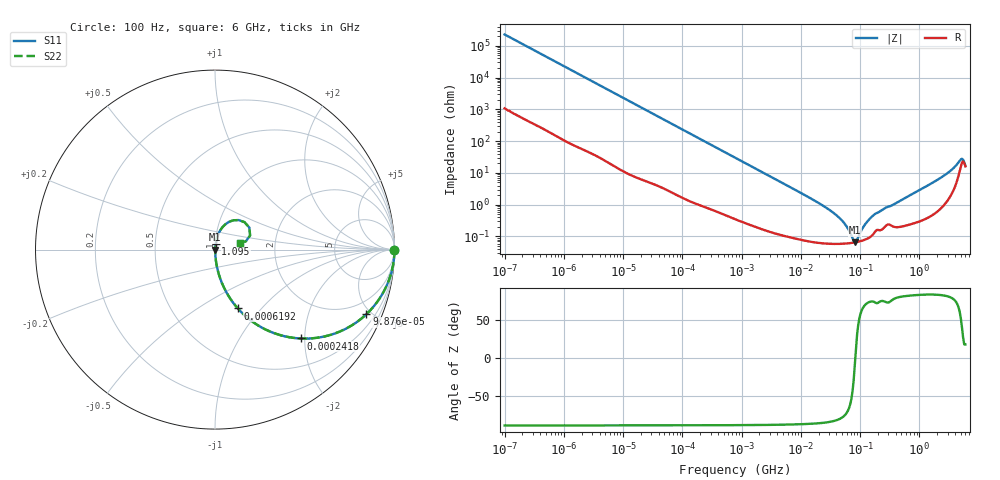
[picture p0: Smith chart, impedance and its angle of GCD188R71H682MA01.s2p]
!Murata Part Number: GCD188R71H682MA01
!These Parameters are Measured in Series Mode Connection
!Data Generated on Mar 13, 2026
!  o--ll--o
!Port1  Port2
!  o------o
!Operation Temp=25[degC], DC Bias Voltage=0[V]
!Freq. Start=100[Hz] Stop=6[GHz] 401[Steps]
# Hz S RI R 50
!Freq.(Hz) S11(Real) S11(Imag) S21(Real) S21(Imag) S12(Real) S12(Imag) S22(Real) S22(Imag)
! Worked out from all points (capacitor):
!   401 points, 100 Hz to 6 GHz, reference 50 ohm
!   read as one part in series: C = 7.03 nF near 109 Hz
!   lowest |Z| = 65.9 mohm at 81.54 MHz (marker M1)
!   series resonance near 83.08 MHz, so ESL is about 520 pH
!   S11 on the Smith chart (normalised r, x): 100 Hz: open; 98.76 kHz: 1.03, -4.68; 241.8 kHz: 1.02, -1.92; 619.2 kHz: 1.01, -0.75; 1.095 GHz: 1.01, +0.06; 6 GHz: 1.32, +0.10
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100  1 -0.000442  2.3e-06 0.000442  2.3e-06 0.000442  1 -0.000442
2008  0.9999 -0.0088  0.000121 0.0088  0.000121 0.0088  0.9999 -0.0088
12592  0.9967 -0.0547  0.00327 0.0547  0.00327 0.0547  0.9967 -0.0547
40335  0.9692 -0.1695  0.0308 0.1695  0.0308 0.1695  0.9692 -0.1695
98762  0.844 -0.3593  0.156 0.3593  0.156 0.3593  0.844 -0.3593
241822  0.4797 -0.4953  0.5203 0.4953  0.5203 0.4953  0.4797 -0.4953
619225  0.1271 -0.3277  0.8729 0.3277  0.8729 0.3277  0.1271 -0.3277
774597  0.0861 -0.2748  0.9139 0.2748  0.9139 0.2748  0.0861 -0.2748
2594782  0.00965 -0.0897  0.9903 0.0897  0.9903 0.0897  0.00965 -0.0897
1.555665e7  0.00089 -0.0148  0.9991 0.0148  0.9991 0.0148  0.00089 -0.0148
4.556224e7  0.000599 -0.00368  0.9994 0.00368  0.9994 0.00368  0.000599 -0.00368
5.960426e7  0.000606 -0.00195  0.9994 0.00195  0.9994 0.00195  0.000606 -0.00195
8.154455e7  0.00065 -0.000106  0.9994 0.000106  0.9994 0.000106  0.00065 -0.000106
8.918374e7  0.000672 0.000412  0.9993 -0.000412  0.9993 -0.000412  0.000672 0.000412
1.166697e8  0.000776 0.00201  0.9992 -0.00201  0.9992 -0.00201  0.000776 0.00201
1.526266e8  0.00102 0.00379  0.999 -0.00379  0.999 -0.00379  0.00102 0.00379
3.124326e8  0.00243 0.00844  0.9976 -0.00844  0.9976 -0.00844  0.00243 0.00844
1.094528e9  0.0041 0.031  0.9959 -0.031  0.9959 -0.031  0.0041 0.031
3.352442e9  0.0304 0.1089  0.9696 -0.1089  0.9696 -0.1089  0.0304 0.1089
4.796499e9  0.1319 0.1644  0.8681 -0.1644  0.8681 -0.1644  0.1319 0.1644
5.245841e9  0.1915 0.1225  0.8085 -0.1225  0.8085 -0.1225  0.1915 0.1225
6e9  0.1403 0.0389  0.8597 -0.0389  0.8597 -0.0389  0.1403 0.0389
